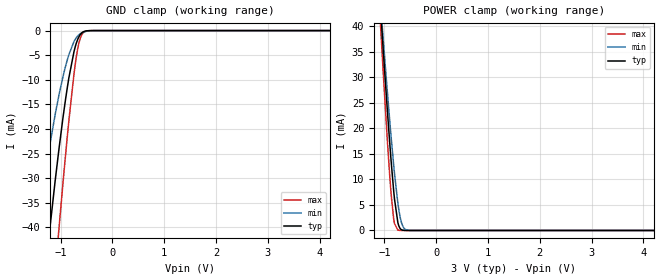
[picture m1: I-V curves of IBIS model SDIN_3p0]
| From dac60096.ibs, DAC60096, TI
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|   Model
[Model]   SDIN_3p0
Model_type   Input
Vinl = 0.21
Vinh = 2.1
|   typ   min   max
C_comp   16.3pF   16.3pF   16.3pF
[Voltage Range]   3   2.999   3.001
[Temperature Range]   27   105   -40
[Power Clamp Reference]   3   2.999   3.001
[GND Clamp Reference]   0   0   0
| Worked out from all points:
|   GND clamp passes 1 mA (typ) near -0.63 V on its own axis
|   POWER clamp passes 1 mA (typ) near -0.72 V on its own axis
[GND Clamp]
|   Voltage   I(typ)   I(min)   I(max)
-3V       -245.1mA   -178.6mA   -302.8mA
-1.461V   -66mA      -40.43mA   -95.45mA
-1.227V   -42.02mA   -24.35mA   -64.76mA
-1.038V   -24.56mA   -13.4mA    -40.95mA
-957mV    -17.89mA   -9.465mA   -31.25mA
-876mV    -11.92mA   -6.12mA    -22.06mA
-741mV    -4.221mA   -2.211mA   -8.71mA
-696mV    -2.531mA   -1.429mA   -5.274mA
-651mV    -1.348mA   -889.7uA   -2.722mA
-606mV    -622uA     -539.9uA   -1.163mA
-552mV    -201.5uA   -283.3uA   -351.2uA
6V        0A         0A         0A
[POWER Clamp]
|   Voltage   I(typ)   I(min)   I(max)
-3V       363.3mA    321.4mA    408.7mA
-1.092V   45.99mA    46.65mA    43.24mA
-1.02V    34.93mA    37.08mA    30.54mA
-930mV    21.71mA    25.55mA    15.64mA
-867mV    13.22mA    17.96mA    6.785mA
-813mV    6.978mA    12mA       1.808mA
-741mV    1.608mA    5.432mA    98.31uA
-696mV    398.6uA    2.616mA    14.66uA
-651mV    79.73uA    995.3uA    2.629uA
-606mV    14.97uA    308.7uA    493.8nA
-525mV    629.8nA    29.46uA    0A
6V        0A         0A         0A
